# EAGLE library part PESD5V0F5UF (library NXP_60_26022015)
Femtofarad unidirectional fivefold ESD protection array Femtofarad capacitance unidirectional ElectroStatic Discharge (ESD) protection diode array designed to protect up to five signal lines from the damage caused by ESD and other transients. The device is encapsulated in a leadless ultra small DFN1410-6 (SOT886) Surface-Mounted Device (SMD) plastic package. The combination of extremely low capacitance, high ESD maximum rating and ultra small package makes the device ideal for high-speed data line protection and antenna protection applications. AAL Eindhoven MK
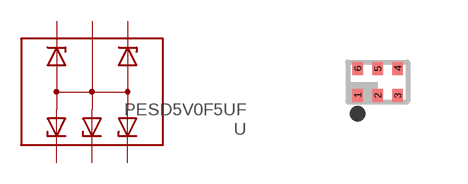
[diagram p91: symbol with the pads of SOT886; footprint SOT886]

Designator prefix U

## PESD5V0F5UF  [SOT886]
1  K1  pas
2  CA  pas
3  K2  pas
4  K3  pas
5  K4  pas
6  K5  pas

## Footprint SOT886 (pad centres in mm)
SOT886 XSON6: plastic extremely thin small outline package; no leads; 6 terminals; body 1 x 1.45 x 0.5 mm JEDEC: MO-252 IEC: ---
smd 0.27 x 0.325: 1 -0.5,-0.338; 2 0,-0.338; 3 0.5,-0.338; 4 0.5,0.338; 5 0,0.338; 6 -0.5,0.338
